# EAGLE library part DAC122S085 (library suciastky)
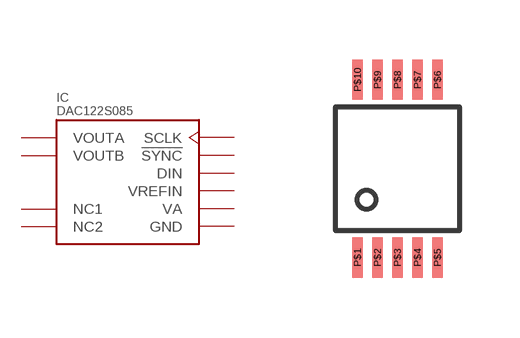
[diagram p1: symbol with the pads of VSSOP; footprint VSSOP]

Designator prefix IC

## DAC122S085  [VSSOP]
P$1  VA  pwr
P$2  VOUTA  out
P$3  VOUTB  out
P$4  NC1  nc
P$5  NC2  nc
P$6  GND  pwr
P$7  VREFIN  in
P$8  DIN
P$9  !SYNC
P$10  SCLK

## Footprint VSSOP (pad centres in mm)
smd 0.254 x 1: P$1 -1,-2.225; P$2 -0.5,-2.225; P$3 0,-2.225; P$4 0.5,-2.225; P$5 1,-2.225; P$6 1,2.225; P$7 0.5,2.225; P$8 0,2.225; P$9 -0.5,2.225; P$10 -1,2.225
